FUNCTION_BLOCK FB_LN_IED_LD1_MMXU1 EXTENDS FB_AcsiCommonLogicalNodeClass
VAR_INPUT
	Beh: FB_DO_IED_LD1_MMXU1_Beh := (sClass:='ENS', bLinkResult:=THIS^.AddDataToContainer(ipData:=Beh));
	PhV: FB_DO_IED_LD1_MMXU1_PhV := (sClass:='WYE', bLinkResult:=THIS^.AddDataToContainer(ipData:=PhV));
END_VAR
VAR
END_VAR

END_FUNCTION_BLOCK
